FUNCTION "Temperature" : VOID
TITLE =
VERSION : 0.1


VAR_TEMP
  TEMPMAX : INT ;
  TEMPMIN : INT ;
END_VAR
BEGIN
NETWORK
TITLE =LETTURA TEMPERATURE STAGNO

      UN    "OFF";
      =     L      4.0;
      U     L      4.0;
      SPBNB _001;
      L     "TC524";
      L     10;
      /I    ;
      T     "DBTemperature".TempAttu[1];
      UN    OV;
      SAVE  ;
      CLR   ;
_001: U     BIE;
      =     L      4.1;
      U     L      4.1;
      SPBNB _002;
      L     "DBTemperature".TempSet[1];
      L     20;
      -I    ;
      T     "DBTemperature".TempSogliaMin[1];
_002: NOP   0;
      U     L      4.1;
      SPBNB _003;
      L     "DBTemperature".TempSet[1];
      L     20;
      +I    ;
      T     "DBTemperature".TempSogliaMax[1];
_003: NOP   0;
      U     L      4.0;
      SPBNB _004;
      L     "TC526";
      L     10;
      /I    ;
      T     "DBTemperature".TempAttu[3];
_004: NOP   0;
      U     L      4.0;
      SPBNB _005;
      L     "TC528";
      L     10;
      /I    ;
      T     "DBTemperature".TempAttu[2];
      UN    OV;
      SAVE  ;
      CLR   ;
_005: U     BIE;
      =     L      4.1;
      U     L      4.1;
      SPBNB _006;
      L     "DBTemperature".TempSet[2];
      L     20;
      -I    ;
      T     "DBTemperature".TempSogliaMin[2];
_006: NOP   0;
      U     L      4.1;
      SPBNB _007;
      L     "DBTemperature".TempSet[2];
      L     20;
      +I    ;
      T     "DBTemperature".TempSogliaMax[2];
_007: NOP   0;
      U     L      4.0;
      SPBNB _008;
      L     "TC530";
      L     10;
      /I    ;
      T     "DBTemperature".TempAttu[4];
_008: NOP   0;
NETWORK
TITLE =ABILITAZIONE RISCALDO VASCA STAGNO 1 E 2

      U     M     56.0;
      =     L      4.0;
      U     L      4.0;
      UN    T     69;
      L     S5T#3S;
      SE    T     68;
      NOP   0;
      NOP   0;
      NOP   0;
      U     T     68;
      L     S5T#7S;
      SE    T     69;
      U(    ;
      U     L      4.0;
      SPBNB _009;
      L     "DBTemperature".TempSet[1];
      L     -2;
      +I    ;
      T     #TEMPMIN;
      UN    OV;
      SAVE  ;
      CLR   ;
_009: U     BIE;
      )     ;
      SPBNB _00a;
      L     "DBTemperature".TempSet[1];
      L     2;
      +I    ;
      T     #TEMPMAX;
_00a: NOP   0;
      U     L      4.0;
      U(    ;
      L     "DBTemperature".TempAttu[1];
      L     #TEMPMIN;
      <I    ;
      )     ;
      U(    ;
      L     "DBTemperature".TempAttu[3];
      L     "DBTemperature".TempSet[1];
      <I    ;
      )     ;
      L     S5T#5S;
      SE    T     70;
      U     L      4.0;
      U(    ;
      O     T     70;
      O     ;
      U(    ;
      L     "DBTemperature".TempAttu[1];
      L     #TEMPMAX;
      <I    ;
      )     ;
      U     T     68;
      )     ;
      =     "ARVS1";
      U(    ;
      U     L      4.0;
      SPBNB _00b;
      L     "DBTemperature".TempSet[2];
      L     -2;
      +I    ;
      T     #TEMPMIN;
      UN    OV;
      SAVE  ;
      CLR   ;
_00b: U     BIE;
      )     ;
      SPBNB _00c;
      L     "DBTemperature".TempSet[2];
      L     2;
      +I    ;
      T     #TEMPMAX;
_00c: NOP   0;
      U     L      4.0;
      U(    ;
      L     "DBTemperature".TempAttu[2];
      L     #TEMPMIN;
      <I    ;
      )     ;
      U(    ;
      L     "DBTemperature".TempAttu[4];
      L     "DBTemperature".TempSet[2];
      <I    ;
      )     ;
      L     S5T#5S;
      SE    T     71;
      U     L      4.0;
      U(    ;
      O     T     71;
      O     ;
      U(    ;
      L     "DBTemperature".TempAttu[2];
      L     #TEMPMAX;
      <I    ;
      )     ;
      U     T     68;
      )     ;
      =     "ARVS2";
NETWORK
TITLE =LETTURA TEMPERATURE STAMPO
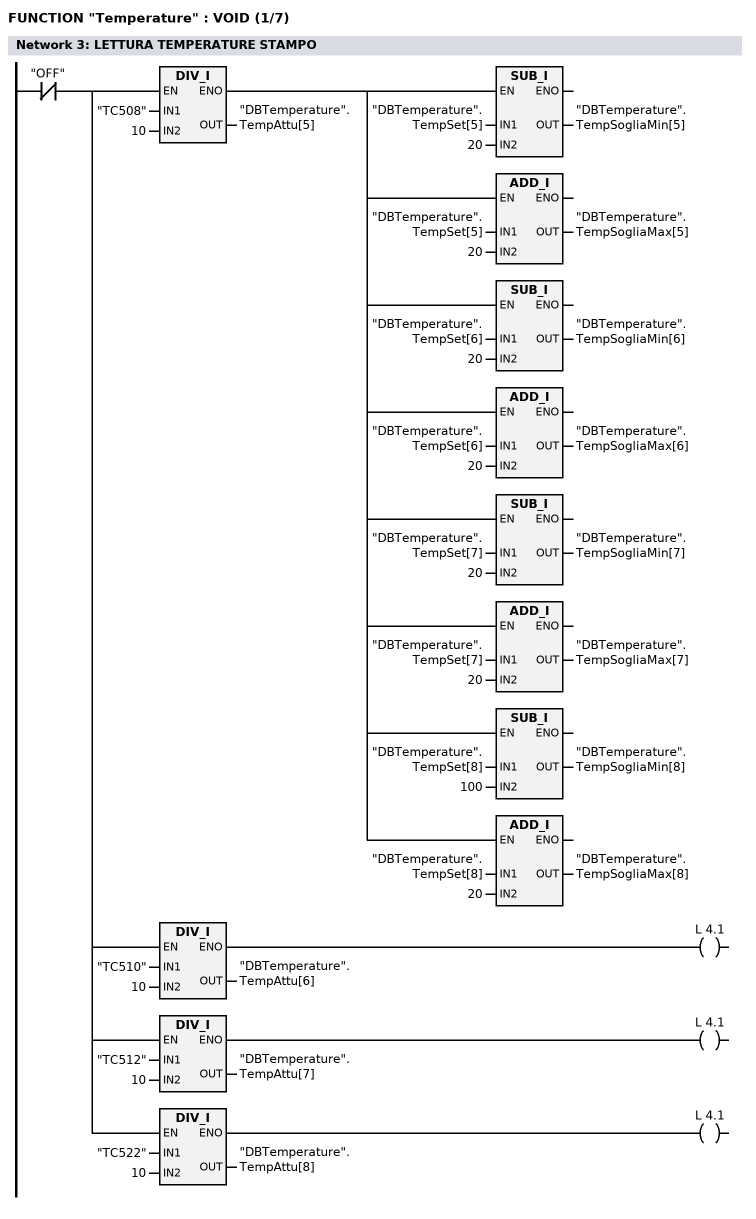
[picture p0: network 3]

      UN    "OFF";
      =     L      4.0;
      U     L      4.0;
      SPBNB _00d;
      L     "TC508";
      L     10;
      /I    ;
      T     "DBTemperature".TempAttu[5];
      UN    OV;
      SAVE  ;
      CLR   ;
_00d: U     BIE;
      =     L      4.1;
      U     L      4.1;
      SPBNB _00e;
      L     "DBTemperature".TempSet[5];
      L     20;
      -I    ;
      T     "DBTemperature".TempSogliaMin[5];
_00e: NOP   0;
      U     L      4.1;
      SPBNB _00f;
      L     "DBTemperature".TempSet[5];
      L     20;
      +I    ;
      T     "DBTemperature".TempSogliaMax[5];
_00f: NOP   0;
      U     L      4.0;
      SPBNB _010;
      L     "TC510";
      L     10;
      /I    ;
      T     "DBTemperature".TempAttu[6];
      UN    OV;
      SAVE  ;
      CLR   ;
_010: U     BIE;
      =     L      4.1;
      U     L      4.1;
      SPBNB _011;
      L     "DBTemperature".TempSet[6];
      L     20;
      -I    ;
      T     "DBTemperature".TempSogliaMin[6];
_011: NOP   0;
      U     L      4.1;
      SPBNB _012;
      L     "DBTemperature".TempSet[6];
      L     20;
      +I    ;
      T     "DBTemperature".TempSogliaMax[6];
_012: NOP   0;
      U     L      4.0;
      SPBNB _013;
      L     "TC512";
      L     10;
      /I    ;
      T     "DBTemperature".TempAttu[7];
      UN    OV;
      SAVE  ;
      CLR   ;
_013: U     BIE;
      =     L      4.1;
      U     L      4.1;
      SPBNB _014;
      L     "DBTemperature".TempSet[7];
      L     20;
      -I    ;
      T     "DBTemperature".TempSogliaMin[7];
_014: NOP   0;
      U     L      4.1;
      SPBNB _015;
      L     "DBTemperature".TempSet[7];
      L     20;
      +I    ;
      T     "DBTemperature".TempSogliaMax[7];
_015: NOP   0;
      U     L      4.0;
      SPBNB _016;
      L     "TC522";
      L     10;
      /I    ;
      T     "DBTemperature".TempAttu[8];
      UN    OV;
      SAVE  ;
      CLR   ;
_016: U     BIE;
      =     L      4.1;
      U     L      4.1;
      SPBNB _017;
      L     "DBTemperature".TempSet[8];
      L     100;
      -I    ;
      T     "DBTemperature".TempSogliaMin[8];
_017: NOP   0;
      U     L      4.1;
      SPBNB _018;
      L     "DBTemperature".TempSet[8];
      L     20;
      +I    ;
      T     "DBTemperature".TempSogliaMax[8];
_018: NOP   0;
NETWORK
TITLE =ABILITAZIONE RISCALDO STAMPO
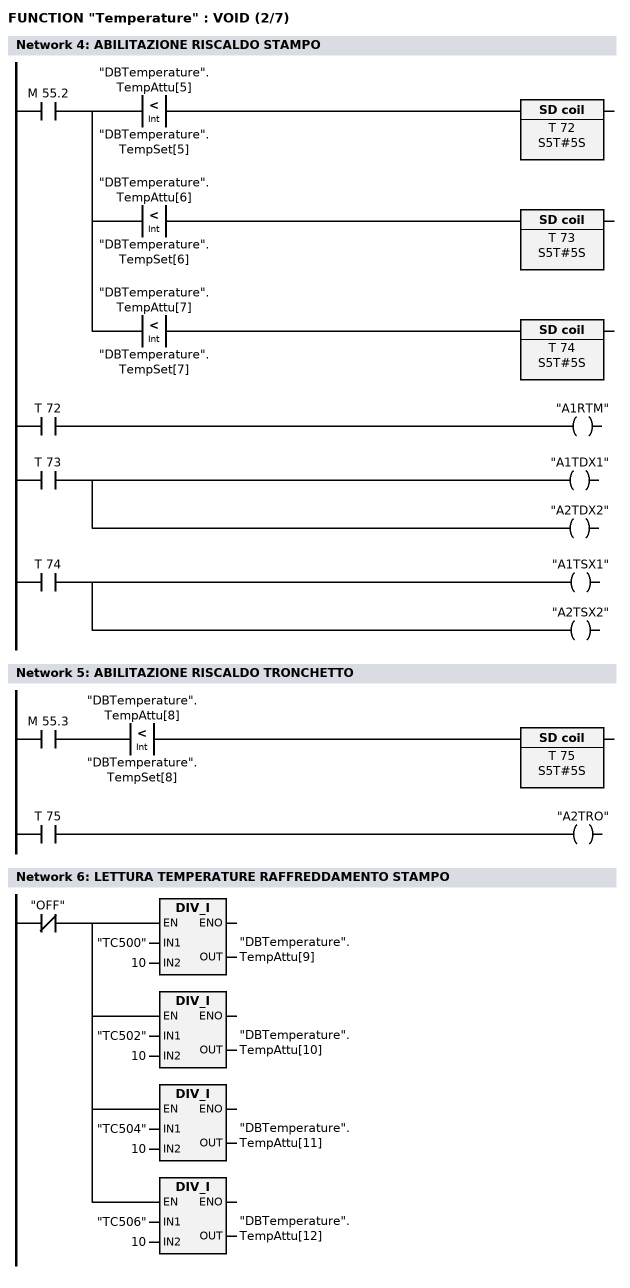
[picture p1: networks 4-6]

      U     M     55.2;
      =     L      4.0;
      U     L      4.0;
      U(    ;
      L     "DBTemperature".TempAttu[5];
      L     "DBTemperature".TempSet[5];
      <I    ;
      )     ;
      L     S5T#5S;
      SE    T     72;
      NOP   0;
      NOP   0;
      NOP   0;
      U     T     72;
      =     "A1RTM";
      U     L      4.0;
      U(    ;
      L     "DBTemperature".TempAttu[6];
      L     "DBTemperature".TempSet[6];
      <I    ;
      )     ;
      L     S5T#5S;
      SE    T     73;
      NOP   0;
      NOP   0;
      NOP   0;
      U     T     73;
      =     "A1TDX1";
      =     "A2TDX2";
      U     L      4.0;
      U(    ;
      L     "DBTemperature".TempAttu[7];
      L     "DBTemperature".TempSet[7];
      <I    ;
      )     ;
      L     S5T#5S;
      SE    T     74;
      NOP   0;
      NOP   0;
      NOP   0;
      U     T     74;
      =     "A1TSX1";
      =     "A2TSX2";
NETWORK
TITLE =ABILITAZIONE RISCALDO TRONCHETTO

      U     M     55.3;
      U(    ;
      L     "DBTemperature".TempAttu[8];
      L     "DBTemperature".TempSet[8];
      <I    ;
      )     ;
      L     S5T#5S;
      SE    T     75;
      NOP   0;
      NOP   0;
      NOP   0;
      U     T     75;
      =     "A2TRO";
NETWORK
TITLE =LETTURA TEMPERATURE RAFFREDDAMENTO STAMPO

      UN    "OFF";
      =     L      4.0;
      U     L      4.0;
      SPBNB _019;
      L     "TC500";
      L     10;
      /I    ;
      T     "DBTemperature".TempAttu[9];
_019: NOP   0;
      U     L      4.0;
      SPBNB _01a;
      L     "TC502";
      L     10;
      /I    ;
      T     "DBTemperature".TempAttu[10];
_01a: NOP   0;
      U     L      4.0;
      SPBNB _01b;
      L     "TC504";
      L     10;
      /I    ;
      T     "DBTemperature".TempAttu[11];
_01b: NOP   0;
      U     L      4.0;
      SPBNB _01c;
      L     "TC506";
      L     10;
      /I    ;
      T     "DBTemperature".TempAttu[12];
_01c: NOP   0;
NETWORK
TITLE =LETTURA TEMPERATURE RAFFREDDAMENTO STAMPO POLARI
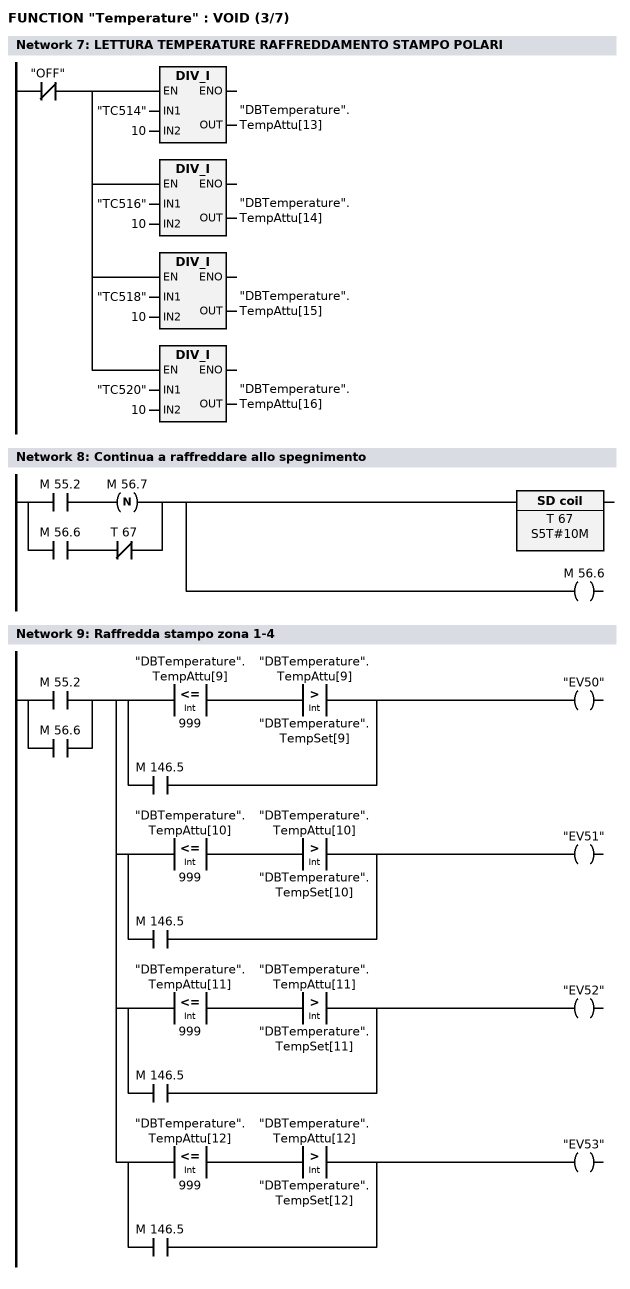
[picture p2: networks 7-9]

      UN    "OFF";
      =     L      4.0;
      U     L      4.0;
      SPBNB _01d;
      L     "TC514";
      L     10;
      /I    ;
      T     "DBTemperature".TempAttu[13];
_01d: NOP   0;
      U     L      4.0;
      SPBNB _01e;
      L     "TC516";
      L     10;
      /I    ;
      T     "DBTemperature".TempAttu[14];
_01e: NOP   0;
      U     L      4.0;
      SPBNB _01f;
      L     "TC518";
      L     10;
      /I    ;
      T     "DBTemperature".TempAttu[15];
_01f: NOP   0;
      U     L      4.0;
      SPBNB _020;
      L     "TC520";
      L     10;
      /I    ;
      T     "DBTemperature".TempAttu[16];
_020: NOP   0;
NETWORK
TITLE =Continua a raffreddare allo spegnimento

      U     M     55.2;
      FN    M     56.7;
      O     ;
      U     M     56.6;
      UN    T     67;
      L     S5T#10M;
      SE    T     67;
      =     M     56.6;
NETWORK
TITLE =Raffredda stampo zona 1-4

      O     M     55.2;
      O     M     56.6;
      =     L      4.0;
      U     L      4.0;
      U(    ;
      U(    ;
      L     "DBTemperature".TempAttu[9];
      L     999;
      <=I   ;
      )     ;
      U(    ;
      L     "DBTemperature".TempAttu[9];
      L     "DBTemperature".TempSet[9];
      >I    ;
      )     ;
      O     M    146.5;
      )     ;
      =     "EV50";
      U     L      4.0;
      U(    ;
      U(    ;
      L     "DBTemperature".TempAttu[10];
      L     999;
      <=I   ;
      )     ;
      U(    ;
      L     "DBTemperature".TempAttu[10];
      L     "DBTemperature".TempSet[10];
      >I    ;
      )     ;
      O     M    146.5;
      )     ;
      =     "EV51";
      U     L      4.0;
      U(    ;
      U(    ;
      L     "DBTemperature".TempAttu[11];
      L     999;
      <=I   ;
      )     ;
      U(    ;
      L     "DBTemperature".TempAttu[11];
      L     "DBTemperature".TempSet[11];
      >I    ;
      )     ;
      O     M    146.5;
      )     ;
      =     "EV52";
      U     L      4.0;
      U(    ;
      U(    ;
      L     "DBTemperature".TempAttu[12];
      L     999;
      <=I   ;
      )     ;
      U(    ;
      L     "DBTemperature".TempAttu[12];
      L     "DBTemperature".TempSet[12];
      >I    ;
      )     ;
      O     M    146.5;
      )     ;
      =     "EV53";
NETWORK
TITLE =Raffredda stampo polari 1-4
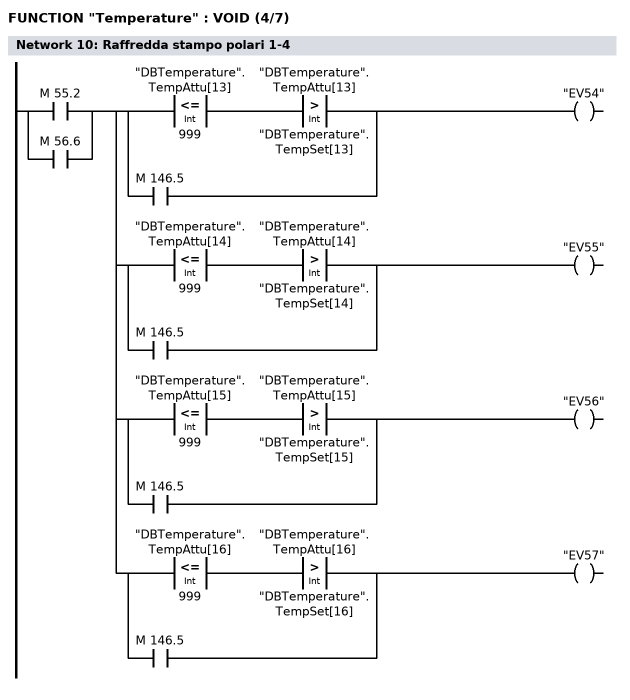
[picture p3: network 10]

      O     M     55.2;
      O     M     56.6;
      =     L      4.0;
      U     L      4.0;
      U(    ;
      U(    ;
      L     "DBTemperature".TempAttu[13];
      L     999;
      <=I   ;
      )     ;
      U(    ;
      L     "DBTemperature".TempAttu[13];
      L     "DBTemperature".TempSet[13];
      >I    ;
      )     ;
      O     M    146.5;
      )     ;
      =     "EV54";
      U     L      4.0;
      U(    ;
      U(    ;
      L     "DBTemperature".TempAttu[14];
      L     999;
      <=I   ;
      )     ;
      U(    ;
      L     "DBTemperature".TempAttu[14];
      L     "DBTemperature".TempSet[14];
      >I    ;
      )     ;
      O     M    146.5;
      )     ;
      =     "EV55";
      U     L      4.0;
      U(    ;
      U(    ;
      L     "DBTemperature".TempAttu[15];
      L     999;
      <=I   ;
      )     ;
      U(    ;
      L     "DBTemperature".TempAttu[15];
      L     "DBTemperature".TempSet[15];
      >I    ;
      )     ;
      O     M    146.5;
      )     ;
      =     "EV56";
      U     L      4.0;
      U(    ;
      U(    ;
      L     "DBTemperature".TempAttu[16];
      L     999;
      <=I   ;
      )     ;
      U(    ;
      L     "DBTemperature".TempAttu[16];
      L     "DBTemperature".TempSet[16];
      >I    ;
      )     ;
      O     M    146.5;
      )     ;
      =     "EV57";
NETWORK
TITLE =Controllo temperatura stagno 1
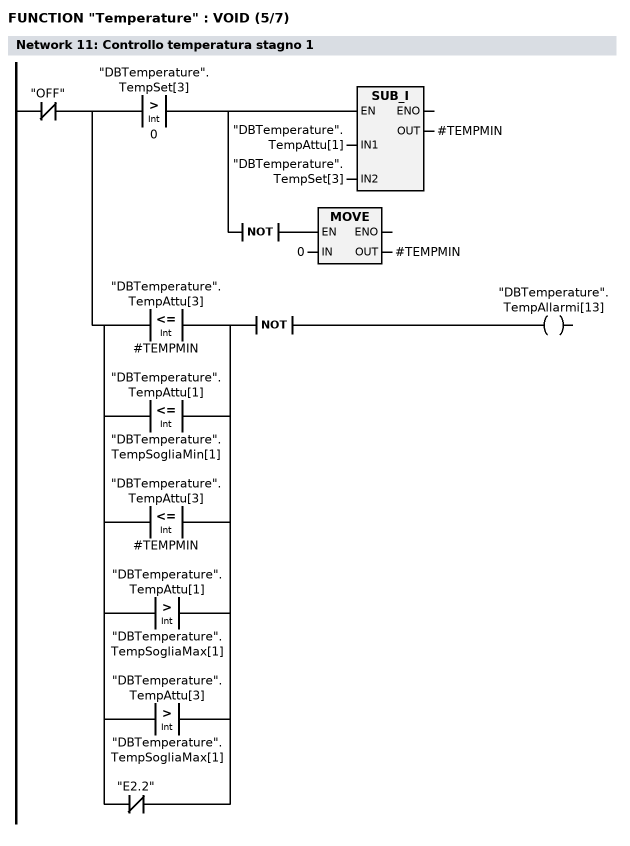
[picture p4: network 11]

      UN    "OFF";
      =     L      4.0;
      U     L      4.0;
      U(    ;
      L     "DBTemperature".TempSet[3];
      L     0;
      >I    ;
      )     ;
      =     L      4.1;
      U     L      4.1;
      SPBNB _021;
      L     "DBTemperature".TempAttu[1];
      L     "DBTemperature".TempSet[3];
      -I    ;
      T     #TEMPMIN;
_021: NOP   0;
      U     L      4.1;
      NOT   ;
      SPBNB _022;
      L     0;
      T     #TEMPMIN;
_022: NOP   0;
      U     L      4.0;
      U(    ;
      O(    ;
      L     "DBTemperature".TempAttu[3];
      L     #TEMPMIN;
      <=I   ;
      )     ;
      O(    ;
      L     "DBTemperature".TempAttu[1];
      L     "DBTemperature".TempSogliaMin[1];
      <=I   ;
      )     ;
      O(    ;
      L     "DBTemperature".TempAttu[3];
      L     #TEMPMIN;
      <=I   ;
      )     ;
      O(    ;
      L     "DBTemperature".TempAttu[1];
      L     "DBTemperature".TempSogliaMax[1];
      >I    ;
      )     ;
      O(    ;
      L     "DBTemperature".TempAttu[3];
      L     "DBTemperature".TempSogliaMax[1];
      >I    ;
      )     ;
      ON    "E2.2";
      )     ;
      NOT   ;
      =     "DBTemperature".TempAllarmi[13];
NETWORK
TITLE =Controllo temperatura stagno 2
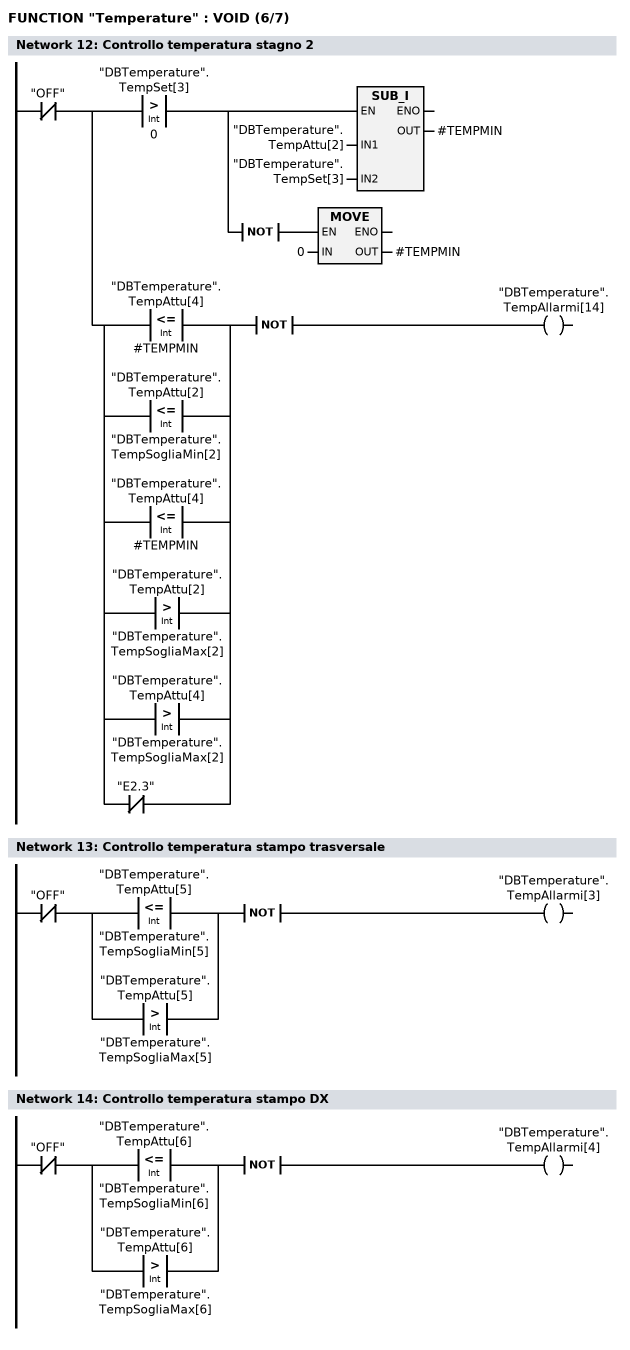
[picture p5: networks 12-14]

      UN    "OFF";
      =     L      4.0;
      U     L      4.0;
      U(    ;
      L     "DBTemperature".TempSet[3];
      L     0;
      >I    ;
      )     ;
      =     L      4.1;
      U     L      4.1;
      SPBNB _023;
      L     "DBTemperature".TempAttu[2];
      L     "DBTemperature".TempSet[3];
      -I    ;
      T     #TEMPMIN;
_023: NOP   0;
      U     L      4.1;
      NOT   ;
      SPBNB _024;
      L     0;
      T     #TEMPMIN;
_024: NOP   0;
      U     L      4.0;
      U(    ;
      O(    ;
      L     "DBTemperature".TempAttu[4];
      L     #TEMPMIN;
      <=I   ;
      )     ;
      O(    ;
      L     "DBTemperature".TempAttu[2];
      L     "DBTemperature".TempSogliaMin[2];
      <=I   ;
      )     ;
      O(    ;
      L     "DBTemperature".TempAttu[4];
      L     #TEMPMIN;
      <=I   ;
      )     ;
      O(    ;
      L     "DBTemperature".TempAttu[2];
      L     "DBTemperature".TempSogliaMax[2];
      >I    ;
      )     ;
      O(    ;
      L     "DBTemperature".TempAttu[4];
      L     "DBTemperature".TempSogliaMax[2];
      >I    ;
      )     ;
      ON    "E2.3";
      )     ;
      NOT   ;
      =     "DBTemperature".TempAllarmi[14];
NETWORK
TITLE =Controllo temperatura stampo trasversale

      UN    "OFF";
      U(    ;
      O(    ;
      L     "DBTemperature".TempAttu[5];
      L     "DBTemperature".TempSogliaMin[5];
      <=I   ;
      )     ;
      O(    ;
      L     "DBTemperature".TempAttu[5];
      L     "DBTemperature".TempSogliaMax[5];
      >I    ;
      )     ;
      )     ;
      NOT   ;
      =     "DBTemperature".TempAllarmi[3];
NETWORK
TITLE =Controllo temperatura stampo DX

      UN    "OFF";
      U(    ;
      O(    ;
      L     "DBTemperature".TempAttu[6];
      L     "DBTemperature".TempSogliaMin[6];
      <=I   ;
      )     ;
      O(    ;
      L     "DBTemperature".TempAttu[6];
      L     "DBTemperature".TempSogliaMax[6];
      >I    ;
      )     ;
      )     ;
      NOT   ;
      =     "DBTemperature".TempAllarmi[4];
NETWORK
TITLE =Controllo temperatura stampo SX
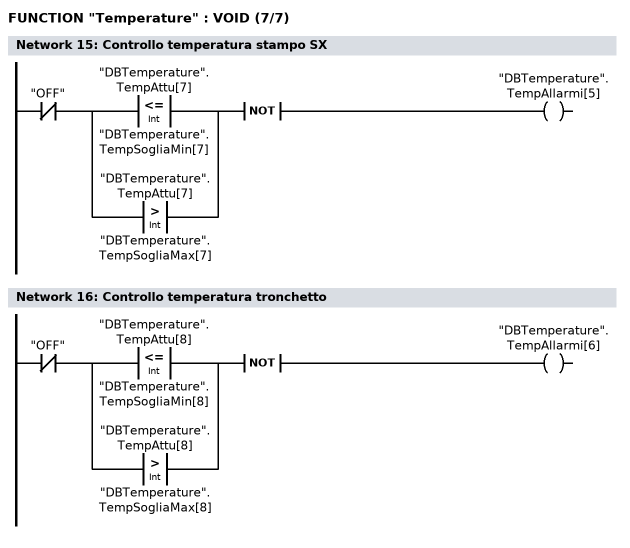
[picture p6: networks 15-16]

      UN    "OFF";
      U(    ;
      O(    ;
      L     "DBTemperature".TempAttu[7];
      L     "DBTemperature".TempSogliaMin[7];
      <=I   ;
      )     ;
      O(    ;
      L     "DBTemperature".TempAttu[7];
      L     "DBTemperature".TempSogliaMax[7];
      >I    ;
      )     ;
      )     ;
      NOT   ;
      =     "DBTemperature".TempAllarmi[5];
NETWORK
TITLE =Controllo temperatura tronchetto

      UN    "OFF";
      U(    ;
      O(    ;
      L     "DBTemperature".TempAttu[8];
      L     "DBTemperature".TempSogliaMin[8];
      <=I   ;
      )     ;
      O(    ;
      L     "DBTemperature".TempAttu[8];
      L     "DBTemperature".TempSogliaMax[8];
      >I    ;
      )     ;
      )     ;
      NOT   ;
      =     "DBTemperature".TempAllarmi[6];
END_FUNCTION

